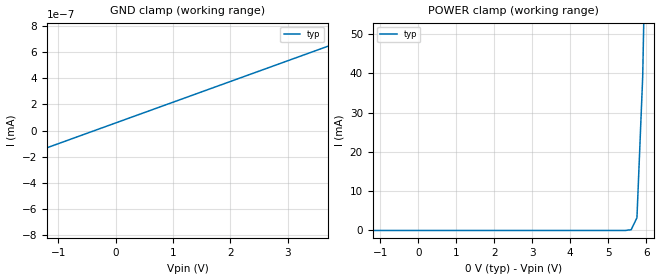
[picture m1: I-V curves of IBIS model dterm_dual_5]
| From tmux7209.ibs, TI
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| dterm_dual_5
[Model]   dterm_dual_5
Model_type   Terminator
|   typ   min   max
C_comp   2.533030e-11   NA   NA
[Voltage Range]   0   -5   5
[Temperature Range]   27   NA   NA
[Power Clamp Reference]   0   NA   NA
[GND Clamp Reference]   0   NA   NA
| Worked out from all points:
|   GND clamp passes 1 mA (typ) near -5.64 V on its own axis
[GND Clamp]
|   Voltage   I(typ)   I(min)   I(max)
-10V      -4.575A    NA         NA
-5.152V   -1.463nA   NA         NA
-5V       -740.1pA   NA         NA
-4.848V   -713.7pA   NA         NA
4.545V    782.9pA    NA         NA
4.697V    807.6pA    NA         NA
5V        858.5pA    NA         NA
[POWER Clamp]
|   Voltage   I(typ)   I(min)   I(max)
-5V       -740.1pA   NA         NA
5.455V    2.806uA    NA         NA
5.606V    199.6uA    NA         NA
5.758V    3.242mA    NA         NA
5.909V    39.13mA    NA         NA
6.061V    114.5mA    NA         NA
10V       5.386A     NA         NA
